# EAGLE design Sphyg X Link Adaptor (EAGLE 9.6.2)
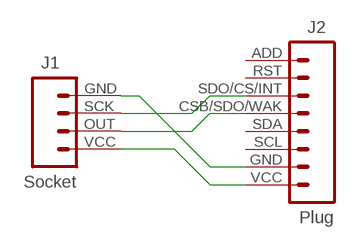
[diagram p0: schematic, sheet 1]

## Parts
J1  Socket  HEADER-1X4-SHPYG  [CONN_04-SPHYG]
J2  Plug  HEADER-1X8-ALF4ALL-SENSOR  [CONN_08-SENSOR]

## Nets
N$1: J1.OUT J2.CSB/SDO/WAK
N$2: J1.SCK J2.SDO/CS/INT
N$4: J1.VCC J2.VCC
N$7: J1.GND J2.GND
Unconnected: J2.ADD J2.RST J2.SCL J2.SDA

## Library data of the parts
J1 = digitalconcepts:HEADER-1X4-SHPYG: Sphygmomanometer Module 4-Pin Header
J2 = digitalconcepts:HEADER-1X8-ALF4ALL-SENSOR: IoT Sensors 1x8 Pin Header for 'Sandwich' IoT Sensors

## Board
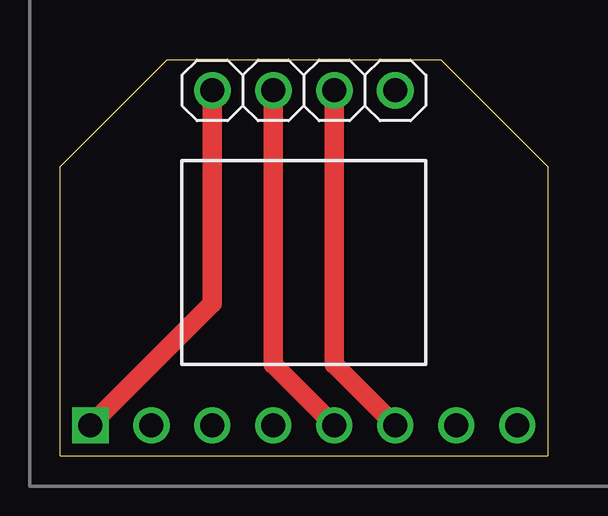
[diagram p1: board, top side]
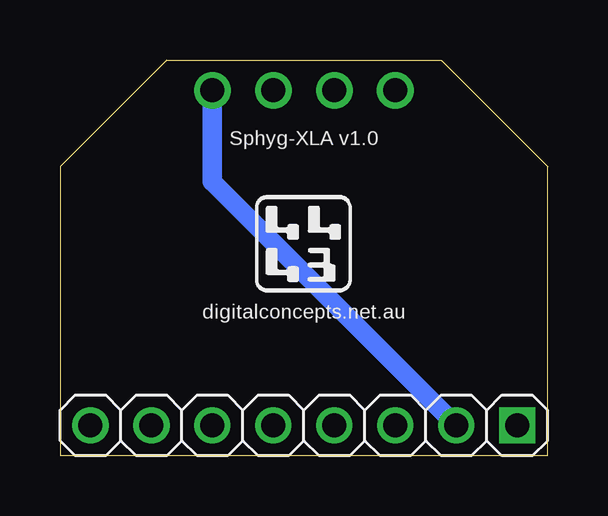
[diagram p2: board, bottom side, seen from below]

Size 20.32 x 16.51 mm. Coordinates in mm from the lower left corner, seen from the top.
Outline: 0,0 20.32,0 20.32,12.07 15.88,16.51 4.45,16.51 0,12.07 0,0
Copper layers (1*16): Top 0.035mm / dielectric 1.5mm / Bottom 0.035mm
Design rules "default *": minimum track width 6mil, minimum drill 0.35mm, track to track 6mil, track to pad 6mil, pad to pad 6mil, via to via 6mil, smd to smd 6mil, copper to edge 15mil, drill to drill 6mil, minimum pad ring 10mil, minimum via ring 8mil, stop-mask expansion 4mil, vias tented up to drill 0mil, thermal gap 10mil

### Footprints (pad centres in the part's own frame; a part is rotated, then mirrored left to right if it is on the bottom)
CONN_04-SPHYG = drill 1 pad 1.524: GND 7.62,0; OUT 2.54,0; SCK 5.08,0; VCC 0,0
CONN_08-SENSOR = drill 1: ADD 17.78,0; CSB/SDO/WAK 10.16,0; GND 2.54,0; RST 15.24,0; SCL 5.08,0; SDA 7.62,0; SDO/CS/INT 12.7,0 | drill 1 square: VCC 0,0

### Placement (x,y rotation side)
J1  6.35,15.24 0 top
J2  1.27,1.27 180 bottom

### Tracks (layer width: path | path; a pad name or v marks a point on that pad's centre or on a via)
N$1
  Top 0.813: J2.CSB/SDO/WAK 8.89,3.81 J1.OUT
N$2
  Top 0.813: J1.SCK 11.43,3.81 J2.SDO/CS/INT
N$4
  Top 0.813: J1.VCC 6.35,6.35 J2.VCC
N$7
  Bottom 0.813: J1.GND 13.97,11.43 J2.GND

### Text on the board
bPlace: Sphyg-XLA v1.0 | digitalconcepts.net.au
